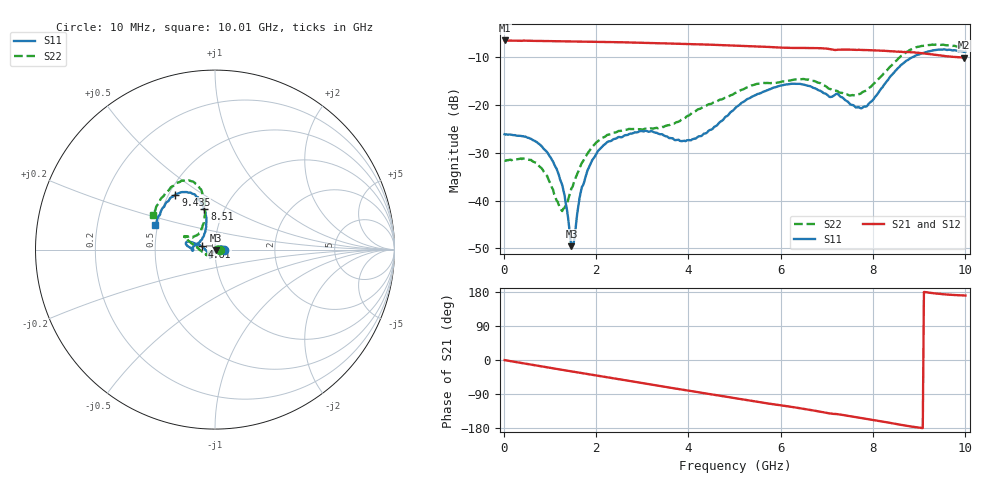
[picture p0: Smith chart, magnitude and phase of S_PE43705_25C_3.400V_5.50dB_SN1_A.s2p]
! Device ID: PE43705
! Serial: 1
! Insertion: A
! Impedance: 50 ohm
! Temp: 25C
! VDD: 3.400V
! Attenuation Step: 5.50dB
#  Hz  S  RI  R  50
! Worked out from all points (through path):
!   401 points, 10 MHz to 10.01 GHz, reference 50 ohm
!   highest |S21| = -6.53 dB at 10 MHz (marker M1); lowest = -10.1 dB at 9.985 GHz (marker M2)
!   group delay of S21, straight-line fit = 54.2 ps
!   lowest |S11| = -49.5 dB at 1.46 GHz (marker M3), VSWR 1.01, Z = 50.3 - j0.161 ohm
!   |S11| at or under -10 dB: start of sweep to 8.869 GHz
!   |S22| runs from -42.2 to -7.4 dB; largest |S21 - S12| = 0.0044
!   S11 on the Smith chart (normalised r, x): 10 MHz: 1.10, -0.00; 4.81 GHz: 0.86, +0.03; 8.51 GHz: 0.81, +0.38; 9.435 GHz: 0.54, +0.39; 10.01 GHz: 0.48, +0.15
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1e7  0.0494 -6.57e-05  0.4713 -0.00223  0.4718 -0.00221  0.0263 9.89e-05
6.35e8  0.0387 0.0177  0.4541 -0.1068  0.4541 -0.1067  0.0185 0.0175
9.85e8  0.0248 0.0154  0.4352 -0.1623  0.4352 -0.1622  0.00666 0.0142
1.26e9  0.0129 0.00681  0.4156 -0.2025  0.4159 -0.2023  -0.00441 0.00641
1.46e9  0.00293 -0.0016  0.3991 -0.2308  0.3992 -0.2307  -0.0134 -0.00114
1.51e9  0.001 -0.00353  0.3944 -0.2379  0.3946 -0.2377  -0.0151 -0.00291
1.685e9  -0.00678 -0.012  0.378 -0.2608  0.378 -0.2607  -0.0225 -0.0104
1.885e9  -0.0143 -0.0203  0.3573 -0.2857  0.3575 -0.2855  -0.0301 -0.018
2.21e9  -0.0214 -0.0335  0.3201 -0.3227  0.3203 -0.3225  -0.0386 -0.0275
3.36e9  -0.0264 -0.0422  0.1634 -0.4093  0.164 -0.4089  -0.0516 -0.0253
4.085e9  -0.0406 -0.0163  0.056 -0.4273  0.0564 -0.4272  -0.0834 -0.00345
4.81e9  -0.0734 0.0174  -0.0502 -0.4163  -0.0495 -0.4165  -0.1165 0.0241
5.01e9  -0.0881 0.0267  -0.0776 -0.4088  -0.0773 -0.4092  -0.1287 0.0336
5.985e9  -0.1522 0.0444  -0.1941 -0.3466  -0.1923 -0.347  -0.1597 0.0664
6.685e9  -0.1518 0.0186  -0.2656 -0.2888  -0.2655 -0.2888  -0.1623 0.0745
7.76e9  -0.0719 0.058  -0.3355 -0.1677  -0.3343 -0.1689  -0.0765 0.11
8.36e9  -0.0496 0.1855  -0.3535 -0.0899  -0.3524 -0.0918  -0.0563 0.24
8.51e9  -0.0594 0.2241  -0.3535 -0.0676  -0.3521 -0.0704  -0.0622 0.283
8.935e9  -0.1137 0.3085  -0.3522 -0.0161  -0.3498 -0.0148  -0.124 0.3796
9.435e9  -0.2208 0.3069  -0.3284 0.0304  -0.3272 0.0307  -0.2217 0.3648
9.985e9  -0.3259 0.1475  -0.308 0.0532  -0.3085 0.0529  -0.338 0.2052
1.001e10  -0.3332 0.1382  -0.3088 0.0538  -0.3104 0.0532  -0.3458 0.1939
